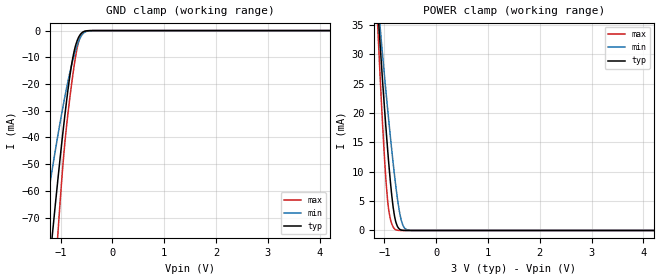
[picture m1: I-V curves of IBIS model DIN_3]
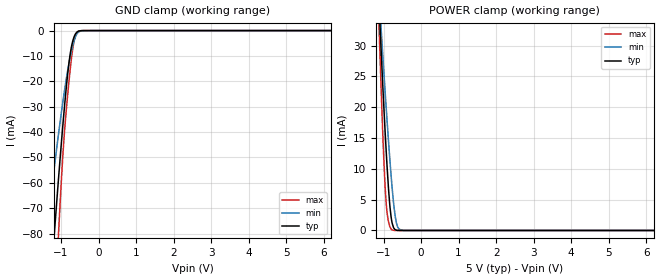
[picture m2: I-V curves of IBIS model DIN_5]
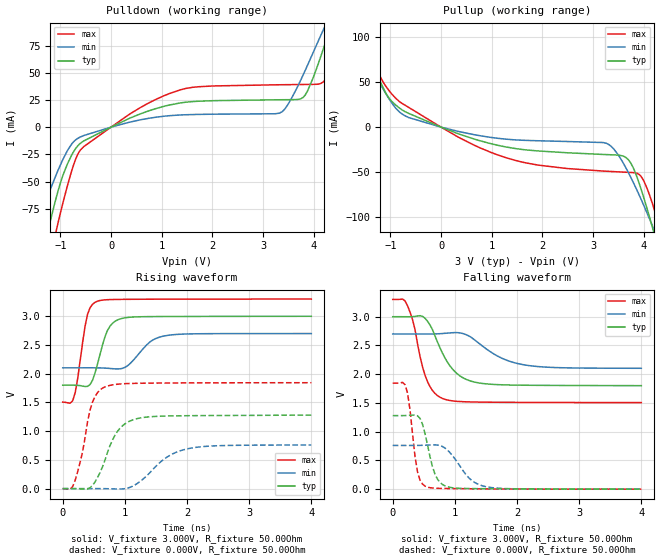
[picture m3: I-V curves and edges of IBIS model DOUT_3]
|Texas Instruments Incorporated
|Dual, 1MSPS, 16/14/12-Bit, 4x2 or 2x2 Channel,
|Simultaneous Sampling, ANALOG-TO-DIGITAL CONVERTER
| Marketing part#   Digital Voltage Range   Package-type   #pins
|ADS7223SRHBR   2.3 V to 5.5 V   QFN   32
|ADS7223SRHBT   2.3 V to 5.5 V   QFN   32
|ADS7263SRHBR   2.3 V to 5.5 V   QFN   32
|ADS7263SRHBT   2.3 V to 5.5 V   QFN   32
|ADS8363SRHBR   2.3 V to 5.5 V   QFN   32
|ADS8363SRHBT   2.3 V to 5.5 V   QFN   32
[IBIS Ver]   4.0
[File name]   ads8363_7263_7223.ibs
[File Rev]   1.0
[Date]   03/17/2010
[Source]   Texas Instruments Incorporated.
   Analog-eLab, HPA
   12500 TI Blvd
   Dallas, TX -75243
   For Support e-mail: elab_ibis@list.ti.com
[Notes]   Revision History:
   1.0: 03/17/2010
   - Initial version of the model
   - Initial Model generated from simulations in TISPICED
   - Model names with a trailing _3 contains the model for
   3V (2.7V and 3.3V). Model names with trailing _5 contains
   the model for 5V (4.75V and 5.25V) operation.
   - Model not matched to measurements
   - min C_comp was obtained at corner high BVDD, low  temperature, strong process
   - max C_comp was obtained at corner low  BVDD, high temperature, weak process
   2.0: 11/08/2010
   - Combined all products (ADS8363, ADS7263, ADS7223) in family into one IBIS
   model.
[Disclaimer]
 This product is designed as an aid for customers of Texas Instruments.
 No warranties, either expressed or implied, with respect to this third
 party software (if any) or with respect to its fitness for any
 particular purpose is claimed by Texas Instruments or the author. The
 software (if any) is provided solely on an "as is" basis. The entire
 risk as to its quality and performance is with the customer
[Copyright] (C) Copyright 2010 Texas Instruments Incorporated.
   All rights reserved.
|   ADS8363. ADS7263 and ADS7223
[Component]   ads8363_7263_7223rhb
[Manufacturer] TI
[Package]
| variable   typ   min   max
R_pkg  0.055614   0.000840   0.081720
L_pkg  0.970664nH 0.141790nH 1.361230nH
C_pkg  0.161895pF 0.102280pF 0.217230pF
[Pin] signal_name  model_name  R_pin  L_pin C_pin
1   CHB1P_CHB2   TERM   0.07117  1.17852nH  0.15277pF
2   CHB1M_CHB1   TERM   0.06724  1.10465nH  0.16414pF
3   CHB0P_CHB0   TERM   0.06702  1.10001nH  0.16329pF
4   CHB0M_CMB   TERM   0.06657  1.09223nH  0.16385pF
5   CHA1P_CHA2   TERM   0.06855  1.12571nH  0.16610pF
6   CHA1M_CHA1   TERM   0.07086  1.16538nH  0.16813pF
7   CHA0P_CHA0   TERM   0.07391  1.21879nH  0.17266pF
8   CHA0M_CMA   TERM   0.08172  1.36123nH  0.16500pF
9   REFIO   TERM   0.02393  0.78169nH  0.21080pF
10   NC   NC   0.02204  0.72161nH  0.21723pF
11   RGND   GND   0.03026  0.70685nH  0.18970pF
12   AGND   GND   0.02001  0.62191nH  0.20207pF
13   AVDD   POWER   0.03031  0.70354nH  0.18370pF
14   NC   NC   0.00084  0.14179nH  0.10234pF
15   NC   NC   0.00084  0.14281nH  0.10228pF
16   M1   DIN   0.07190  1.18424nH  0.15073pF
17   M0   DIN   0.07319  1.20582nH  0.15450pF
18   SDI   DIN   0.06804  1.11035nH  0.16610pF
19   CONVST   DIN   0.06721  1.09512nH  0.16502pF
20   RD   DIN   0.07012  1.14509nH  0.16621pF
21   _CS   DIN   0.07014  1.14529nH  0.16623pF
22   CLOCK   DIN   0.06721  1.09510nH  0.16504pF
23   BUSY   DOUT   0.06804  1.11039nH  0.16613pF
24   SDOB   DOUT   0.07317  1.20553nH  0.15454pF
25   SDOA   DOUT   0.07187  1.18372nH  0.15183pF
26   NC   NC   0.00084  0.14279nH  0.10231pF
27   BVDD   POWER   0.05954  0.97215nH  0.15618pF
28   BGND   GND   0.06498  1.06373nH  0.16191pF
29   AVDD   POWER   0.06239  1.02006nH  0.15850pF
30   AGND   GND   0.06597  1.08097nH  0.16200pF
31   NC   NC   0.06067  0.99231nH  0.15775pF
32   NC   NC   0.06909  1.14187nH  0.15159pF
|   Model Selectors
[Model Selector]   DIN
DIN_3   2.70V - 3.30V Input Model
DIN_5   4.50V - 5.50V Input Model
[Model Selector]   DOUT
DOUT_3   2.70V - 3.30V Output Model
DOUT_5   4.50V - 5.50V Output Model
|   TERM Model
[Model] TERM
Model_type Terminator
C_comp   0   0   0
| variable   typ   min   max
[Voltage Range]   3.3V   2.0V   5.5V
[POWER Clamp Reference]  3.3V   2.0V   5.5V
[GND Clamp Reference]   0.0V   0.0V   0.0V
|Operating Temperature
[Temperature Range]   27   125   -40
| Models and submodels in the file (5): TERM (Terminator), DIN_3 (Input), DIN_5 (Input), DOUT_3 (Output), DOUT_5 (Output)
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|   INPUT 3.0V model
[Model]   DIN_3
Model_type   Input
| Signals   M0, M1, SDI, CONVST, RD, _SC, CLOCK, BUSY
Vinl = 900.000mV
Vinh = 2.1V
| C_comp   obtained at 25MHz
| variable   typ   min   max
C_comp   3.806pF   2.861pF   4.719pF
[Temperature Range]   40.0   125.0   -40.0
[Voltage range]   3.0V   2.7V   3.3V
[power clamp reference] 3.0V   2.7V   3.3V
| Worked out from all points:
|   GND clamp passes 1 mA (typ) near -0.60 V on its own axis
|   POWER clamp passes 1 mA (typ) near -0.76 V on its own axis
[GND Clamp]
|   Voltage   I(typ)   I(min)   I(max)
-3V       -493.1mA   -328.5mA   -702.2mA
-1.383V   -122.5mA   -79.89mA   -177.4mA
-1.326V   -110.4mA   -72.39mA   -159.3mA
-1.179V   -80.14mA   -53.91mA   -113.4mA
-1.121V   -68.8mA    -47.05mA   -96.04mA
-1.054V   -55.86mA   -39.26mA   -76.29mA
-917.6mV  -31.58mA   -24.69mA   -41.86mA
-787.1mV  -12.59mA   -12.82mA   -19.83mA
-721.9mV  -6.351mA   -8.03mA    -10.97mA
-660mV    -2.796mA   -4.418mA   -4.757mA
-549.8mV  -340.5uA   -799.5uA   -408.9uA
5.999V    0A         0A         0A
[POWER Clamp]
|   Voltage   I(typ)   I(min)   I(max)
-3V       226.3mA    192mA      270.5mA
-1.136V   38.85mA    40.03mA    35.99mA
-1.107V   34.88mA    37.04mA    30.59mA
-1.072V   30.23mA    33.52mA    24.33mA
-996.4mV  20.62mA    26.16mA    12.09mA
-939mV    13.94mA    20.82mA    5.225mA
-910.9mV  10.94mA    18.28mA    3.164mA
-845.6mV  5.024mA    12.67mA    875.5uA
-773.6mV  1.289mA    7.125mA    95.94uA
-656.6mV  44.02uA    1.217mA    1.965uA
-494.6mV  190nA      16.18uA    -23.79nA
5.999V    -35.58nA   -43.76nA   -28.45nA
|   INPUT 5.0V Model
[Model]   DIN_5
Model_type   Input
| Signals   M0, M1, SDI, CONVST, RD, _SC, CLOCK, BUSY
Vinl = 1.5V
Vinh = 3.5V
| C_comp   obtained at 25MHz
| variable   typ   min   max
C_comp   3.408pF   2.584pF   4.227pF
[Temperature Range]   40.0   125.0   -40.0
[Voltage range]   5.0V   4.50V   5.50V
[power clamp reference] 5.0V   4.50V   5.50V
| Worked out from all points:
|   GND clamp passes 1 mA (typ) near -0.60 V on its own axis
|   POWER clamp passes 1 mA (typ) near -0.76 V on its own axis
[GND Clamp]
|   Voltage   I(typ)   I(min)   I(max)
-5V       -965.7mA   -668.8mA   -1.352A
-1.402V   -126.5mA   -82.34mA   -183.3mA
-1.312V   -107.4mA   -70.57mA   -154.8mA
-1.166V   -77.55mA   -52.34mA   -109.4mA
-1.094V   -63.6mA    -43.91mA   -88.07mA
-1.053V   -55.75mA   -39.19mA   -76.11mA
-968.8mV  -40.35mA   -29.96mA   -53.42mA
-914.4mV  -31.04mA   -24.37mA   -41.2mA
-771.9mV  -10.89mA   -11.62mA   -17.61mA
-651.9mV  -2.469mA   -4.02mA    -4.15mA
-522.5mV  -179.9uA   -465.9uA   -188.1uA
9.998V    0A         0A         0A
[POWER Clamp]
|   Voltage   I(typ)   I(min)   I(max)
-5V       320.7mA    274.7mA    381.2mA
-1.117V   36.27mA    38.08mA    32.47mA
-1.055V   28.03mA    31.85mA    21.43mA
-1.001V   21.14mA    26.56mA    12.71mA
-953.8mV  15.6mA     22.17mA    6.678mA
-914.4mV  11.3mA     18.6mA     3.371mA
-869.4mV  6.963mA    14.67mA    1.459mA
-828.1mV  3.801mA    11.25mA    561.2uA
-770mV    1.186mA    6.872mA    84.49uA
-657.5mV  45.3uA     1.24mA     2.004uA
-485mV    108nA      12.27uA    43.95nA
9.998V    0A         0A         0A
|   Output 3.0V Model
[Model]   DOUT_3
Model_type   Output
|Signals   SDOA, SDOB
Vmeas = 1.523V
Cref = 30.00pF
| C_comp   obtained at 36MHz
| variable   typ   min   max
|C_comp Output Low
C_comp   4.178pF   3.202pF   5.099pF
|C_comp Output High
|C_comp   4.247pF   3.275pF   5.243pF
[Model Spec]
Vmeas   1.52V   1.34V   1.77V
Vref   2.50V   0.50V   3.00V
|Junction Temperature
[Temperature Range]   40.0   125.0   -40.0
[Voltage range]   3.0V   2.70V   3.3V
[Pullup reference]   3.0V   2.7V   3.3V
[power clamp reference]   3.0V   2.7V   3.3V
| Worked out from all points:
|   slope of the pulldown table from 0 to 0.45 V, typ, clamps not added: 46.1 ohm
|   slope of the pullup table from 0 to 0.45 V, typ, clamps not added: 47.6 ohm
|   falling waveform, V_fixture 3.000V, R_fixture 50.00Ohm: 20-80 % time 359ps typ, 552ps min, 242ps max; typ from 3 V to 1.8 V
|   rising waveform, V_fixture 3.000V, R_fixture 50.00Ohm: 20-80 % time 197ps typ, 315ps min, 149ps max; typ from 1.8 V to 3 V
|   rising waveform, V_fixture 0.000V, R_fixture 50.00Ohm: 20-80 % time 312ps typ, 499ps min, 212ps max; typ from 0 V to 1.28 V
|   falling waveform, V_fixture 0.000V, R_fixture 50.00Ohm: 20-80 % time 176ps typ, 329ps min, 124ps max; typ from 1.28 V to 0 V
[Pulldown]
|   Voltage   I(typ)   I(min)   I(max)
-3V       -493.5mA   -328.7mA   -702.6mA
-1.482V   -144.9mA   -93.75mA   -210.6mA
-1.222V   -91.05mA   -60.13mA   -130.9mA
-1.074V   -63.32mA   -42.73mA   -93.54mA
-627.4mV  -15.75mA   -9.559mA   -22.54mA
576.4mV   12.15mA    6.695mA    17.93mA
1.473V    22.93mA    11.39mA    35.55mA
3.321V    25.18mA    12.81mA    38.97mA
3.834V    29.57mA    52.23mA    39.24mA
4.231V    77.55mA    93.58mA    44.03mA
4.626V    130.9mA    131.1mA    111.8mA
5.999V    252.7mA    219.9mA    290mA
[Pullup]
|   Voltage   I(typ)   I(min)   I(max)
-3V       226.4mA    192.1mA    270.6mA
-1.885V   136.6mA    115.4mA    166.2mA
-1.55V    96.55mA    83.71mA    114.7mA
-1.175V   47.75mA    45.61mA    53.31mA
-639.8mV  15.32mA    10.68mA    22mA
1.267V    -21.91mA   -13.31mA   -33.75mA
3.309V    -30.66mA   -19.21mA   -49.22mA
3.74V     -39.35mA   -55.1mA    -50.41mA
3.962V    -71.05mA   -81.77mA   -55.79mA
4.175V    -111.8mA   -110mA     -85.27mA
4.301V    -137.8mA   -127.6mA   -113.4mA
5.999V    -527.8mA   -397.6mA   -658.4mA
[Ramp]
R_load = 50.00Ohm
|   typ   min   max
dV/dt_r   767.588mV/312.304ps 456.037mV/498.579ps   1.106V/212.465ps
dV/dt_f   719.581mV/358.502ps 358.322mV/552.147ps   1.076V/241.501ps
[Falling Waveform]
V_fixture = 3.000V
V_fixture_min = 2.700V
V_fixture_max = 3.300V
R_fixture = 50.00Ohm
|   Time   V(typ)   V(min)   V(max)
0s        3V         2.7V       3.3V
240ps     2.999V     2.7V       3.187V
320ps     3.001V     2.7V       2.944V
520ps     2.973V     2.699V     1.983V
640ps     2.774V     2.7V       1.716V
800ps     2.367V     2.708V     1.578V
1.04ns    2.005V     2.723V     1.527V
1.4ns     1.846V     2.527V     1.515V
2.16ns    1.808V     2.155V     1.509V
4ns       1.801V     2.103V     1.507V
[Rising Waveform]
V_fixture = 3.000V
V_fixture_min = 2.700V
V_fixture_max = 3.300V
R_fixture = 50.00Ohm
|   Time   V(typ)   V(min)   V(max)
0s        1.801V     2.103V     1.507V
160ps     1.801V     2.103V     1.53V
240ps     1.798V     2.103V     1.91V
400ps     1.78V      2.103V     3.037V
560ps     2.169V     2.103V     3.263V
720ps     2.753V     2.095V     3.289V
960ps     2.965V     2.093V     3.295V
1.4ns     2.994V     2.55V      3.297V
1.64ns    2.996V     2.659V     3.298V
4ns       3V         2.7V       3.3V
[Rising Waveform]
V_fixture = 0.000V
V_fixture_min = 0.000V
V_fixture_max = 0.000V
R_fixture = 50.00Ohm
|   Time   V(typ)   V(min)   V(max)
0s        -885.7nV   -1.489uV   -525.3nV
160ps     405.1uV    12.3uV     36.11mV
320ps     -6.546mV   181.8uV    640.3mV
480ps     56.17mV    451.2uV    1.507V
680ps     495.9mV    -767.9uV   1.771V
880ps     994.4mV    -6.557mV   1.817V
1.2ns     1.219V     89.63mV    1.833V
1.64ns    1.263V     520.4mV    1.838V
2ns       1.269V     691.1mV    1.84V
4ns       1.279V     760.1mV    1.844V
[Falling Waveform]
V_fixture = 0.000V
V_fixture_min = 0.000V
V_fixture_max = 0.000V
R_fixture = 50.00Ohm
|   Time   V(typ)   V(min)   V(max)
0s        1.279V     760.1mV    1.844V
200ps     1.28V      759.7mV    1.815V
280ps     1.285V     759.7mV    1.364V
400ps     1.276V     760.7mV    294.1mV
520ps     967.7mV    764.8mV    52.82mV
680ps     261mV      770.9mV    16.79mV
880ps     42.01mV    681mV      11.34mV
1.24ns    10.39mV    180.9mV    7.385mV
1.52ns    7.799mV    38.94mV    4.655mV
4ns       -885.7nV   -1.489uV   -525.3nV
